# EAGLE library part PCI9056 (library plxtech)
PCI 9056 PCI Bus Mastering I/O Accelerator between a 32-bit, 66 MHz PCI Bus and 32-bit, 66 MHz processor Local Bus Data Book Version 0.91b February 2002 Website: http://www.plxtech.com
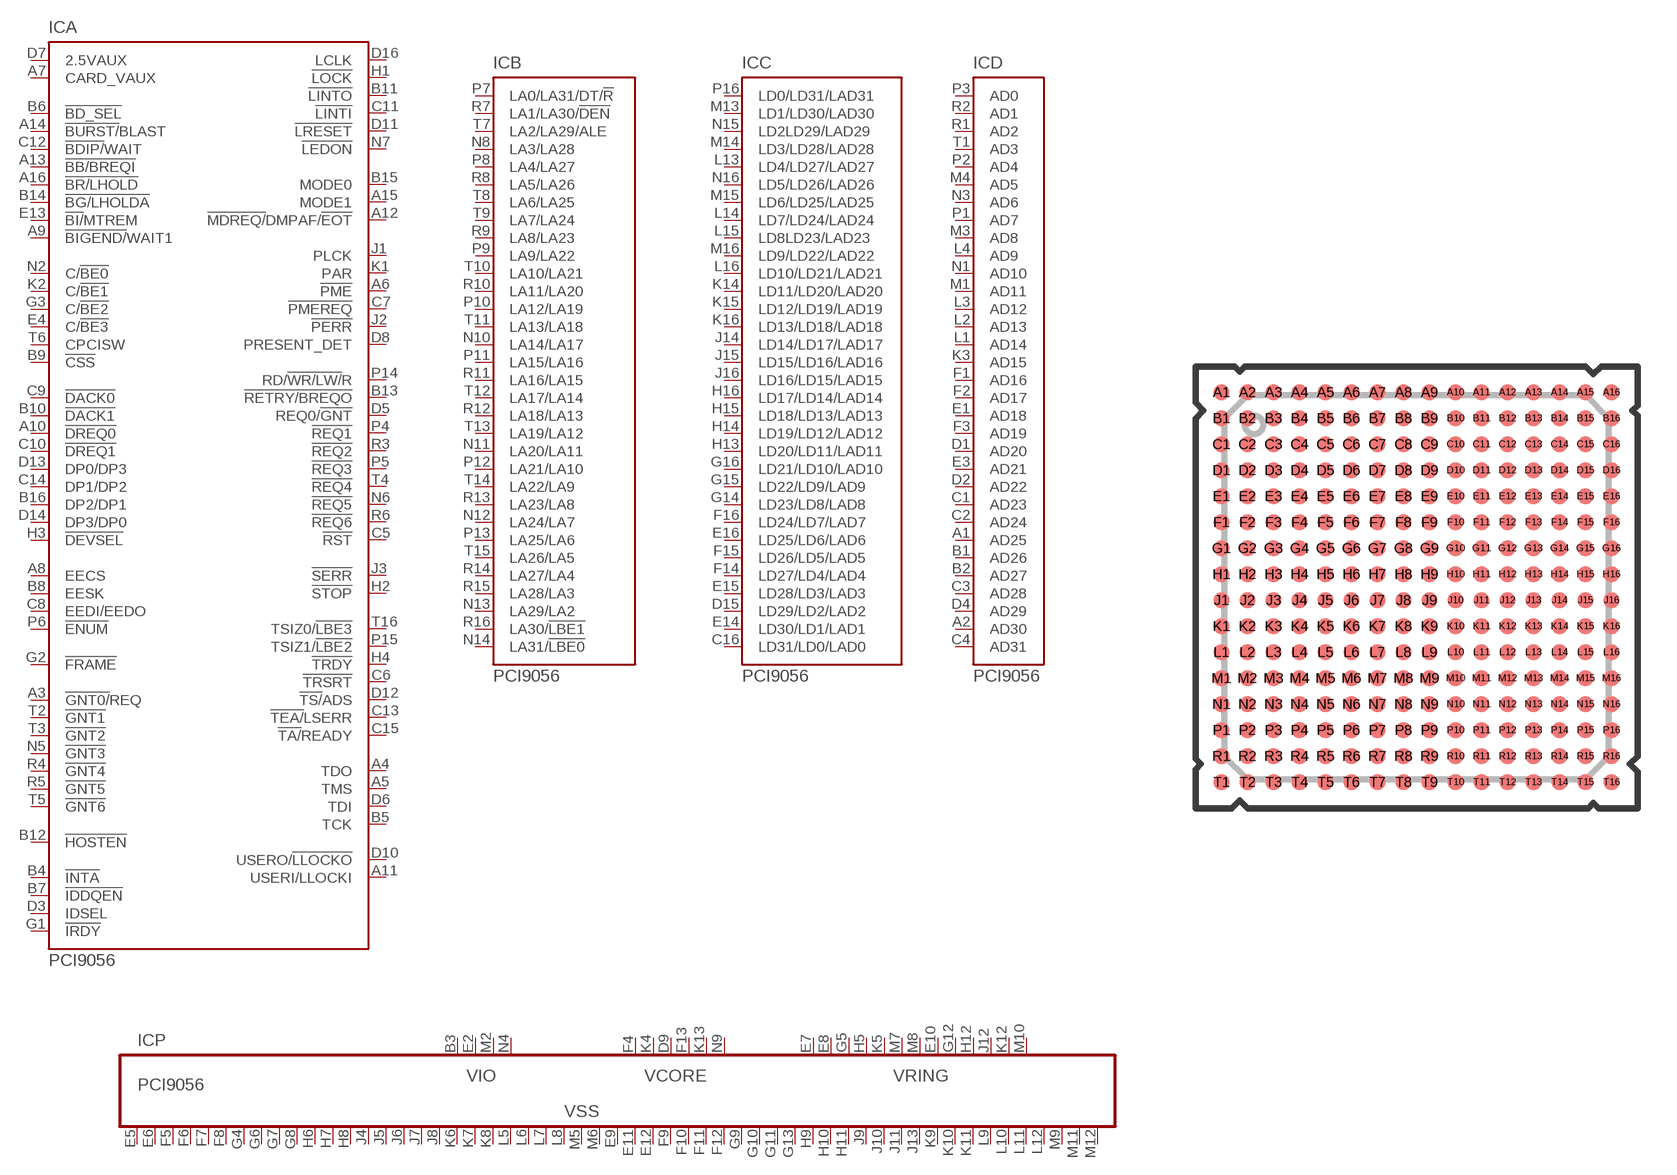
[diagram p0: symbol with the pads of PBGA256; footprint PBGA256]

Designator prefix IC; gates A=PCI9056 B=PCI-LA C=PCI-LD D=PCI-AD P=PWR-PCI9056

## PCI9056 (OC_FARNELL: 1623124; OC_NEWARK: unknown)  [PBGA256]
A1  D:AD25
A2  D:AD30
A3  A:!GNT0/!REQ  out
A4  A:TDO
A5  A:TMS  in
A6  A:!PME
A7  A:CARD_VAUX  pwr
A8  A:EECS  out
A9  A:!BIGEND/!WAIT1
A10  A:!DREQ0  in
A11  A:USERI/LLOCKI  in
A12  A:!MDREQ/!DMPAF/!EOT
A13  A:!BB/BREQI  in
A14  A:!BURST/!BLAST
A15  A:MODE1  in
A16  A:!BR/LHOLD  out
B1  D:AD26
B2  D:AD27
B3  P:VIO  pwr
B4  A:!INTA
B5  A:TCK  in
B6  A:!BD_SEL  in
B7  A:!IDDQEN  in
B8  A:EESK  out
B9  A:!CSS  in
B10  A:!DACK1  out
B11  A:!LINTO  out
B12  A:!HOSTEN  in
B13  A:!RETRY/BREQO  out
B14  A:!BG/LHOLDA  in
B15  A:MODE0  in
B16  A:DP2/DP1
C1  D:AD23
C2  D:AD24
C3  D:AD28
C4  D:AD31
C5  A:!RST
C6  A:!TRSRT  in
C7  A:!PMEREQ  in
C8  A:EEDI/EEDO
C9  A:!DACK0  out
C10  A:!DREQ1  in
C11  A:!LINTI  in
C12  A:!BDIP/!WAIT
C13  A:!TEA/!LSERR
C14  A:DP1/DP2
C15  A:!TA/!READY
C16  C:LD31/LD0/LAD0  in
D1  D:AD20
D2  D:AD22
D3  A:IDSEL  in
D4  D:AD29
D5  A:REQ0/!GNT  in
D6  A:TDI  in
D7  A:2.5VAUX  pwr
D8  A:PRESENT_DET  in
D9  P:VCORE  pwr
D10  A:USERO/!LLOCKO
D11  A:!LRESET
D12  A:!TS/!ADS
D13  A:DP0/DP3
D14  A:DP3/DP0
D15  C:LD29/LD2/LAD2  in
D16  A:LCLK  in
E1  D:AD18
E2  P:VIO  pwr
E3  D:AD21
E4  A:C/!BE3
E5  P:VSS  pwr
E6  P:VSS  pwr
E7  P:VRING  pwr
E8  P:VRING  pwr
E9  P:VSS  pwr
E10  P:VRING  pwr
E11  P:VSS  pwr
E12  P:VSS  pwr
E13  A:!BI/!MTREM  in
E14  C:LD30/LD1/LAD1  in
E15  C:LD28/LD3/LAD3  in
E16  C:LD25/LD6/LAD6  in
F1  D:AD16
F2  D:AD17
F3  D:AD19
F4  P:VCORE  pwr
F5  P:VSS  pwr
F6  P:VSS  pwr
F7  P:VSS  pwr
F8  P:VSS  pwr
F9  P:VSS  pwr
F10  P:VSS  pwr
F11  P:VSS  pwr
F12  P:VSS  pwr
F13  P:VCORE  pwr
F14  C:LD27/LD4/LAD4  in
F15  C:LD26/LD5/LAD5  in
F16  C:LD24/LD7/LAD7  in
G1  A:!IRDY
G2  A:!FRAME
G3  A:C/!BE2
G4  P:VSS  pwr
G5  P:VRING  pwr
G6  P:VSS  pwr
G7  P:VSS  pwr
G8  P:VSS  pwr
G9  P:VSS  pwr
G10  P:VSS  pwr
G11  P:VSS  pwr
G12  P:VRING  pwr
G13  P:VSS  pwr
G14  C:LD23/LD8/LAD8  in
G15  C:LD22/LD9/LAD9  in
G16  C:LD21/LD10/LAD10  in
H1  A:!LOCK
H2  A:!STOP
H3  A:!DEVSEL
H4  A:!TRDY
H5  P:VRING  pwr
H6  P:VSS  pwr
H7  P:VSS  pwr
H8  P:VSS  pwr
H9  P:VSS  pwr
H10  P:VSS  pwr
H11  P:VSS  pwr
H12  P:VRING  pwr
H13  C:LD20/LD11/LAD11  in
H14  C:LD19/LD12/LAD12  in
H15  C:LD18/LD13/LAD13  in
H16  C:LD17/LD14/LAD14  in
J1  A:PLCK  in
J2  A:!PERR
J3  A:!SERR
J4  P:VSS  pwr
J5  P:VSS  pwr
J6  P:VSS  pwr
J7  P:VSS  pwr
J8  P:VSS  pwr
J9  P:VSS  pwr
J10  P:VSS  pwr
J11  P:VSS  pwr
J12  P:VRING  pwr
J13  P:VSS  pwr
J14  C:LD14/LD17/LAD17  in
J15  C:LD15/LD16/LAD16  in
J16  C:LD16/LD15/LAD15  in
K1  A:PAR
K2  A:C/!BE1
K3  D:AD15
K4  P:VCORE  pwr
K5  P:VRING  pwr
K6  P:VSS  pwr
K7  P:VSS  pwr
K8  P:VSS  pwr
K9  P:VSS  pwr
K10  P:VSS  pwr
K11  P:VSS  pwr
K12  P:VRING  pwr
K13  P:VCORE  pwr
K14  C:LD11/LD20/LAD20  in
K15  C:LD12/LD19/LAD19  in
K16  C:LD13/LD18/LAD18  in
L1  D:AD14
L2  D:AD13
L3  D:AD12
L4  D:AD9
L5  P:VSS  pwr
L6  P:VSS  pwr
L7  P:VSS  pwr
L8  P:VSS  pwr
L9  P:VSS  pwr
L10  P:VSS  pwr
L11  P:VSS  pwr
L12  P:VSS  pwr
L13  C:LD4/LD27/LAD27  in
L14  C:LD7/LD24/LAD24  in
L15  C:LD8LD23/LAD23  in
L16  C:LD10/LD21/LAD21  in
M1  D:AD11
M2  P:VIO  pwr
M3  D:AD8
M4  D:AD5
M5  P:VSS  pwr
M6  P:VSS  pwr
M7  P:VRING  pwr
M8  P:VRING  pwr
M9  P:VSS  pwr
M10  P:VRING  pwr
M11  P:VSS  pwr
M12  P:VSS  pwr
M13  C:LD1/LD30/LAD30  in
M14  C:LD3/LD28/LAD28  in
M15  C:LD6/LD25/LAD25  in
M16  C:LD9/LD22/LAD22  in
N1  D:AD10
N2  A:C/!BE0
N3  D:AD6
N4  P:VIO  pwr
N5  A:!GNT3  out
N6  A:!REQ5  in
N7  A:!LEDON  out
N8  B:LA3/LA28  in
N9  P:VCORE  pwr
N10  B:LA14/LA17  in
N11  B:LA20/LA11  in
N12  B:LA24/LA7  in
N13  B:LA29/LA2  in
N14  B:LA31/!LBE0  in
N15  C:LD2LD29/LAD29  in
N16  C:LD5/LD26/LAD26  in
P1  D:AD7
P2  D:AD4
P3  D:AD0
P4  A:!REQ1  in
P5  A:!REQ3  in
P6  A:!ENUM  out
P7  B:LA0/LA31/DT/!R  in
P8  B:LA4/LA27  in
P9  B:LA9/LA22  in
P10  B:LA12/LA19  in
P11  B:LA15/LA16  in
P12  B:LA21/LA10  in
P13  B:LA25/LA6  in
P14  A:RD/!WR/LW/!R
P15  A:TSIZ1/!LBE2
P16  C:LD0/LD31/LAD31  in
R1  D:AD2
R2  D:AD1
R3  A:!REQ2  in
R4  A:!GNT4  out
R5  A:!GNT5  out
R6  A:!REQ6  in
R7  B:LA1/LA30/!DEN  in
R8  B:LA5/LA26  in
R9  B:LA8/LA23  in
R10  B:LA11/LA20  in
R11  B:LA16/LA15  in
R12  B:LA18/LA13  in
R13  B:LA23/LA8  in
R14  B:LA27/LA4  in
R15  B:LA28/LA3  in
R16  B:LA30/!LBE1  in
T1  D:AD3
T2  A:!GNT1  out
T3  A:!GNT2  out
T4  A:!REQ4  in
T5  A:!GNT6  out
T6  A:CPCISW  in
T7  B:LA2/LA29/ALE  in
T8  B:LA6/LA25  in
T9  B:LA7/LA24  in
T10  B:LA10/LA21  in
T11  B:LA13/LA18  in
T12  B:LA17/LA14  in
T13  B:LA19/LA12  in
T14  B:LA22/LA9  in
T15  B:LA26/LA5  in
T16  A:TSIZ0/!LBE3

## Footprint PBGA256 (pad centres in mm)
Ball Grid Array PBGA 256
smd 0.6 x 0.6: A1 -7.5,7.5; A2 -6.5,7.5; A3 -5.5,7.5; A4 -4.5,7.5; A5 -3.5,7.5; A6 -2.5,7.5; A7 -1.5,7.5; A8 -0.5,7.5; A9 0.5,7.5; A10 1.5,7.5; A11 2.5,7.5; A12 3.5,7.5; A13 4.5,7.5; A14 5.5,7.5; A15 6.5,7.5; A16 7.5,7.5; B1 -7.5,6.5; B2 -6.5,6.5; B3 -5.5,6.5; B4 -4.5,6.5; B5 -3.5,6.5; B6 -2.5,6.5; B7 -1.5,6.5; B8 -0.5,6.5; B9 0.5,6.5; B10 1.5,6.5; B11 2.5,6.5; B12 3.5,6.5; B13 4.5,6.5; B14 5.5,6.5; B15 6.5,6.5; B16 7.5,6.5; C1 -7.5,5.5; C2 -6.5,5.5; C3 -5.5,5.5; C4 -4.5,5.5; C5 -3.5,5.5; C6 -2.5,5.5; C7 -1.5,5.5; C8 -0.5,5.5; C9 0.5,5.5; C10 1.5,5.5; C11 2.5,5.5; C12 3.5,5.5; C13 4.5,5.5; C14 5.5,5.5; C15 6.5,5.5; C16 7.5,5.5; D1 -7.5,4.5; D2 -6.5,4.5; D3 -5.5,4.5; D4 -4.5,4.5; D5 -3.5,4.5; D6 -2.5,4.5; D7 -1.5,4.5; D8 -0.5,4.5; D9 0.5,4.5; D10 1.5,4.5; D11 2.5,4.5; D12 3.5,4.5; D13 4.5,4.5; D14 5.5,4.5; D15 6.5,4.5; D16 7.5,4.5; E1 -7.5,3.5; E2 -6.5,3.5; E3 -5.5,3.5; E4 -4.5,3.5; E5 -3.5,3.5; E6 -2.5,3.5; E7 -1.5,3.5; E8 -0.5,3.5; E9 0.5,3.5; E10 1.5,3.5; E11 2.5,3.5; E12 3.5,3.5; E13 4.5,3.5; E14 5.5,3.5; E15 6.5,3.5; E16 7.5,3.5; F1 -7.5,2.5; F2 -6.5,2.5; F3 -5.5,2.5; F4 -4.5,2.5; F5 -3.5,2.5; F6 -2.5,2.5; F7 -1.5,2.5; F8 -0.5,2.5; F9 0.5,2.5; F10 1.5,2.5; F11 2.5,2.5; F12 3.5,2.5; F13 4.5,2.5; F14 5.5,2.5; F15 6.5,2.5; F16 7.5,2.5; G1 -7.5,1.5; G2 -6.5,1.5; G3 -5.5,1.5; G4 -4.5,1.5; G5 -3.5,1.5; G6 -2.5,1.5; G7 -1.5,1.5; G8 -0.5,1.5; G9 0.5,1.5; G10 1.5,1.5; G11 2.5,1.5; G12 3.5,1.5; G13 4.5,1.5; G14 5.5,1.5; G15 6.5,1.5; G16 7.5,1.5; H1 -7.5,0.5; H2 -6.5,0.5; H3 -5.5,0.5; H4 -4.5,0.5; H5 -3.5,0.5; H6 -2.5,0.5; H7 -1.5,0.5; H8 -0.5,0.5; H9 0.5,0.5; H10 1.5,0.5; H11 2.5,0.5; H12 3.5,0.5; H13 4.5,0.5; H14 5.5,0.5; H15 6.5,0.5; H16 7.5,0.5; J1 -7.5,-0.5; J2 -6.5,-0.5; J3 -5.5,-0.5; J4 -4.5,-0.5; J5 -3.5,-0.5; J6 -2.5,-0.5; J7 -1.5,-0.5; J8 -0.5,-0.5; J9 0.5,-0.5; J10 1.5,-0.5; J11 2.5,-0.5; J12 3.5,-0.5; J13 4.5,-0.5; J14 5.5,-0.5; J15 6.5,-0.5; J16 7.5,-0.5; K1 -7.5,-1.5; K2 -6.5,-1.5; K3 -5.5,-1.5; K4 -4.5,-1.5; K5 -3.5,-1.5; K6 -2.5,-1.5; K7 -1.5,-1.5; K8 -0.5,-1.5; K9 0.5,-1.5; K10 1.5,-1.5; K11 2.5,-1.5; K12 3.5,-1.5; K13 4.5,-1.5; K14 5.5,-1.5; K15 6.5,-1.5; K16 7.5,-1.5; L1 -7.5,-2.5; L2 -6.5,-2.5; L3 -5.5,-2.5; L4 -4.5,-2.5; L5 -3.5,-2.5; L6 -2.5,-2.5; L7 -1.5,-2.5; L8 -0.5,-2.5; L9 0.5,-2.5; L10 1.5,-2.5; L11 2.5,-2.5; L12 3.5,-2.5; L13 4.5,-2.5; L14 5.5,-2.5; L15 6.5,-2.5; L16 7.5,-2.5; M1 -7.5,-3.5; M2 -6.5,-3.5; M3 -5.5,-3.5; M4 -4.5,-3.5; M5 -3.5,-3.5; M6 -2.5,-3.5; M7 -1.5,-3.5; M8 -0.5,-3.5; M9 0.5,-3.5; M10 1.5,-3.5; M11 2.5,-3.5; M12 3.5,-3.5; M13 4.5,-3.5; M14 5.5,-3.5; M15 6.5,-3.5; M16 7.5,-3.5; N1 -7.5,-4.5; N2 -6.5,-4.5; N3 -5.5,-4.5; N4 -4.5,-4.5; N5 -3.5,-4.5; N6 -2.5,-4.5; N7 -1.5,-4.5; N8 -0.5,-4.5; N9 0.5,-4.5; N10 1.5,-4.5; N11 2.5,-4.5; N12 3.5,-4.5; N13 4.5,-4.5; N14 5.5,-4.5; N15 6.5,-4.5; N16 7.5,-4.5; P1 -7.5,-5.5; P2 -6.5,-5.5; P3 -5.5,-5.5; P4 -4.5,-5.5; P5 -3.5,-5.5; P6 -2.5,-5.5; P7 -1.5,-5.5; P8 -0.5,-5.5; P9 0.5,-5.5; P10 1.5,-5.5; P11 2.5,-5.5; P12 3.5,-5.5; P13 4.5,-5.5; P14 5.5,-5.5; P15 6.5,-5.5; P16 7.5,-5.5; R1 -7.5,-6.5; R2 -6.5,-6.5; R3 -5.5,-6.5; R4 -4.5,-6.5; R5 -3.5,-6.5; R6 -2.5,-6.5; R7 -1.5,-6.5; R8 -0.5,-6.5; R9 0.5,-6.5; R10 1.5,-6.5; R11 2.5,-6.5; R12 3.5,-6.5; R13 4.5,-6.5; R14 5.5,-6.5; R15 6.5,-6.5; R16 7.5,-6.5; T1 -7.5,-7.5; T2 -6.5,-7.5; T3 -5.5,-7.5; T4 -4.5,-7.5; T5 -3.5,-7.5; T6 -2.5,-7.5; T7 -1.5,-7.5; T8 -0.5,-7.5; T9 0.5,-7.5; T10 1.5,-7.5; T11 2.5,-7.5; T12 3.5,-7.5; T13 4.5,-7.5; T14 5.5,-7.5; T15 6.5,-7.5; T16 7.5,-7.5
